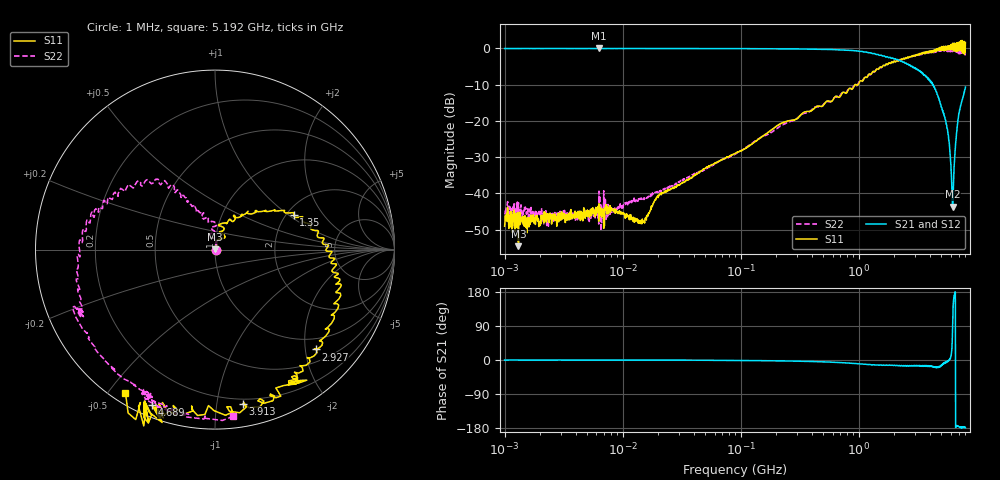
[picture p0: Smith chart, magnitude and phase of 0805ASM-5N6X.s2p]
!s-Parameter Generated by FASTRON Sdn. Bhd.
!FASTRON P/N : 0805ASM-5N6X
!Keysight Technologies: E5071C_MY46733604_B.14.02
!Date: Fri Jun 19 14:46:22 2026
!Version  :Rev00  Fri Jun 19 14:46:22 2026
!Data & Calibration Information:
!Freq  S11:SOLT2(ON)  S21:SOLT2(ON)  S12:SOLT2(ON)  S22:SOLT2(ON)
!PortZ  Port1:50+j0  Port2:50+j0
!When reading reference impedance value at option line is always used.
! Remarks : This data is being provided solely for informational purposes.
# Hz S dB R 50
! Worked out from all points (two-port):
!   1601 points, 1 MHz to 8 GHz, reference 50 ohm
!   highest |S21| = -0.02 dB at 6.301 MHz (marker M1); lowest = -43.7 dB at 6.226 GHz (marker M2)
!   |S21| within 3 dB of the highest: start of sweep to 2.064 GHz
!   lowest |S11| = -54.6 dB at 1.31 MHz (marker M3), VSWR 1.00, Z = 50 + j0.18 ohm
!   |S11| at or under -10 dB: start of sweep to 929.3 MHz; 951.7 MHz to 985.4 MHz (33.69 MHz wide, 3.48 % of centre)
!   |S22| runs from -50.4 to -0.3 dB; largest |S21 - S12| = 0.0079
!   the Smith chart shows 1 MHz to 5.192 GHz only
!   S11 on the Smith chart (normalised r, x): 1 MHz: 1.01, -0.00; 1.35 GHz: 2.19, +1.10; 2.927 GHz: 0.75, -2.21; 3.913 GHz: 0.16, -1.18; 4.689 GHz: 0.05, -0.67; 5.192 GHz: 0.04, -0.55
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1000000  -49.10 -14.6  -0.05 -0.1  -0.05 -0.1  -45.60 0.5
1310238  -54.60 74.7  -0.09 0.1  -0.06 -0.1  -42.60 -20.4
4479405  -46.20 11.9  -0.05 -0.1  -0.05 -0.1  -46.60 18.6
6301378  -42.90 25.8  -0.02 -0.3  -0.03 -0.0  -39.40 34.9
1.46648e7  -47.10 44.2  -0.05 -0.2  -0.06 -0.3  -41.50 39.5
2.00676e7  -40.70 50.6  -0.06 -0.3  -0.07 -0.2  -39.60 57.1
8.994653e7  -29.00 75.7  -0.07 -1.1  -0.09 -1.1  -29.10 77.6
4.006501e8  -17.10 81.4  -0.22 -4.0  -0.22 -4.0  -16.90 87.0
1.349549e9  -6.38 23.8  -1.44 -12.7  -1.45 -12.9  -6.54 130.0
1.7949e9  -4.10 2.5  -2.58 -13.7  -2.58 -14.0  -4.06 147.0
2.472225e9  -2.77 -19.3  -4.14 -15.4  -4.20 -15.5  -2.71 167.0
2.927065e9  -2.05 -44.8  -5.29 -15.8  -5.34 -15.7  -2.16 -168.0
3.912882e9  -1.17 -79.9  -8.67 -17.2  -8.61 -17.2  -1.23 -135.0
4.26866e9  -0.57 -101.0  -9.94 -18.0  -9.96 -18.3  -1.06 -118.0
4.688537e9  -0.58 -112.0  -13.30 -20.0  -13.30 -20.2  -0.80 -112.0
5.192391e9  -0.53 -122.0  -17.90 -11.0  -17.80 -11.0  -0.59 -83.8
5.64026e9  0.62 -138.0  -22.30 -4.1  -22.30 -4.1  -0.59 -59.9
6.033702e9  1.05 -139.0  -32.30 10.6  -32.20 10.2  -0.43 -50.8
6.226476e9  1.39 -135.0  -43.70 82.7  -43.70 81.9  -0.38 -43.2
6.419251e9  1.48 -142.0  -32.70 170.0  -32.80 169.0  -0.53 -27.3
7.036128e9  0.72 -165.0  -18.00 -176.0  -18.10 -176.0  -0.74 16.4
8e9  1.63 158.0  -10.70 -179.0  -10.60 -179.0  -1.03 42.2
